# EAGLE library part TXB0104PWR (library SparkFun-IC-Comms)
4-Bit Bi-Directional Level Shifter 1.2V-3.6V (VCCA) to 1.65V-5.5V (VCCB) bi-directional level shifter with auto direction sensing. Max data rate - VCCA 1.8V: 20Mbps (50ns), VCCA 3.3V: 100Mbps (10ns) Digikey: 296-21929-1-ND (TSSOP) Datasheet SparkFun Products SparkFun Cellular Shield - MG2639 (CEL-13120) SparkFun Level Shifting microSD Breakout (DEV-13743) SparkFun Voltage-Level Translator Breakout - TXB0104 (BOB-11771) SparkFun Block for Intel® Edison - UART (DEV-13040) SparkFun Block for Intel® Edison - Arduino (DEV-13036)
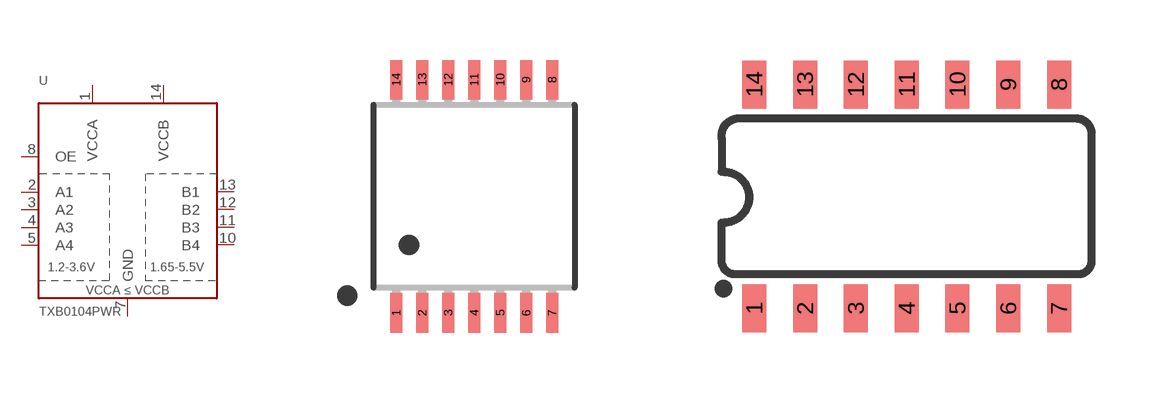
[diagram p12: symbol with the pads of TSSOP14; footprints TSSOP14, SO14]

Designator prefix U

## TXB0104PWR (PROD_ID: IC-13929; VALUE: TXB0104)  [TSSOP14]
1  VCCA
2  A1
3  A2
4  A3
5  A4
7  GND
8  OE
10  B4
11  B3
12  B2
13  B1
14  VCCB

## TXB0104PWRSOIC14 (PROD_ID: IC-11329; VALUE: TXB0104)  [SO14]
Pads as for TSSOP14

## Footprint TSSOP14 (pad centres in mm)
TSSOP (Thin Shrink Small Outline Plastic) - 14 Specifications: Pin count:14 Example device(s): TXB0104PWR
smd 0.305 x 0.991: 1 -1.95,-2.918; 2 -1.3,-2.918; 3 -0.65,-2.918; 4 0,-2.918; 5 0.65,-2.918; 6 1.3,-2.918; 7 1.95,-2.918; 8 1.95,2.918; 9 1.3,2.918; 10 0.65,2.918; 11 0,2.918; 12 -0.65,2.918; 13 -1.3,2.918; 14 -1.95,2.918

## Footprint SO14 (pad centres in mm)
SOIC - 14 Specifications: Pin count:14 Example device(s): TXB0104PWR
smd 0.6 x 1.2: 1 -3.81,-2.8; 2 -2.54,-2.8; 3 -1.27,-2.8; 4 0,-2.8; 5 1.27,-2.8; 6 2.54,-2.8; 7 3.81,-2.8; 8 3.81,2.8; 9 2.54,2.8; 10 1.27,2.8; 11 0,2.8; 12 -1.27,2.8; 13 -2.54,2.8; 14 -3.81,2.8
